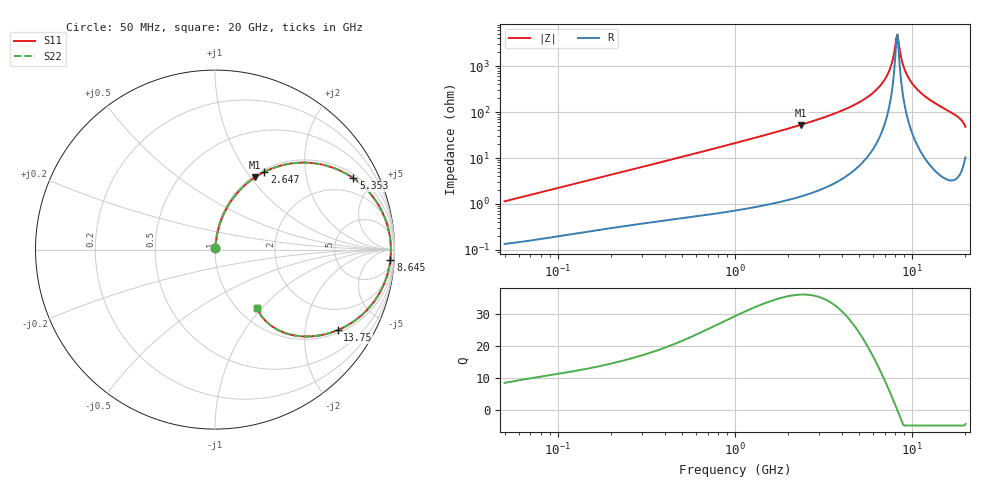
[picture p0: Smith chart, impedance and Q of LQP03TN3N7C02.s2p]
!Murata Part Number: LQP03TN3N7C02
!These Parameters are Measured in Series Mode Connection
!  o--[Z]--o
!Port1  Port2
!  o-------o
!Freq. Start=50[MHz] Stop=20[GHz], 401[Steps]
# Hz S RI R 50
!Freq.(Hz) S11(Real) S11(Imag) S21(Real) S21(Imag) S12(Real) S12(Imag) S22(Real) S22(Imag)
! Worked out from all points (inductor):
!   401 points, 50 MHz to 20 GHz, reference 50 ohm
!   read as one part in series: L = 3.59 nH near 51.52 MHz
!   highest Q = 36.2 at 2.349 GHz (marker M1), where L = 3.56 nH
!   self-resonance near 8.142 GHz
!   S11 on the Smith chart (normalised r, x): 50 MHz: 1.00, +0.02; 2.647 GHz: 1.03, +1.21; 5.353 GHz: 1.17, +3.77; 8.645 GHz: 12, -31; 13.75 GHz: 1.10, -2.98; 20 GHz: 1.21, -0.94
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5e7  0.00148 0.0113  0.9985 -0.0113  0.9985 -0.0113  0.00148 0.0113
1.364002e8  0.00328 0.0298  0.9967 -0.0298  0.9967 -0.0298  0.00328 0.0298
3.721004e8  0.0103 0.0779  0.9897 -0.0779  0.9897 -0.0779  0.0103 0.0779
1e9  0.0488 0.1992  0.9512 -0.1992  0.9512 -0.1992  0.0488 0.1992
2.348516e9  0.2228 0.4026  0.7772 -0.4026  0.7772 -0.4026  0.2228 0.4026
2.647493e9  0.2744 0.4326  0.7256 -0.4326  0.7256 -0.4326  0.2744 0.4326
2.728004e9  0.2889 0.4396  0.7111 -0.4396  0.7111 -0.4396  0.2889 0.4396
3.967106e9  0.5266 0.4835  0.4734 -0.4835  0.4734 -0.4835  0.5266 0.4835
5.352748e9  0.7705 0.3982  0.2295 -0.3982  0.2295 -0.3982  0.7705 0.3982
6.503449e9  0.9079 0.2533  0.0921 -0.2533  0.0921 -0.2533  0.9079 0.2533
7.009217e9  0.9451 0.1797  0.0549 -0.1797  0.0549 -0.1797  0.9451 0.1797
7.442007e9  0.9659 0.1155  0.0341 -0.1155  0.0341 -0.1155  0.9659 0.1155
7.668323e9  0.9729 0.0821  0.0271 -0.0821  0.0271 -0.0821  0.9729 0.0821
8.141811e9  0.98 0.0137  0.02 -0.0137  0.02 -0.0137  0.98 0.0137
8.389408e9  0.9799 -0.0209  0.0201 0.0209  0.0201 0.0209  0.9799 -0.0209
8.644534e9  0.9773 -0.0554  0.0227 0.0554  0.0227 0.0554  0.9773 -0.0554
9.178299e9  0.9648 -0.1235  0.0352 0.1235  0.0352 0.1235  0.9648 -0.1235
1.004137e10  0.9287 -0.2198  0.0713 0.2198  0.0713 0.2198  0.9287 -0.2198
1.149051e10  0.8414 -0.3421  0.1586 0.3421  0.1586 0.3421  0.8414 -0.3421
1.375312e10  0.6839 -0.4488  0.3161 0.4488  0.3161 0.4488  0.6839 -0.4488
1.747767e10  0.4336 -0.4765  0.5664 0.4765  0.5664 0.4765  0.4336 -0.4765
2e10  0.2324 -0.326  0.7676 0.326  0.7676 0.326  0.2324 -0.326
